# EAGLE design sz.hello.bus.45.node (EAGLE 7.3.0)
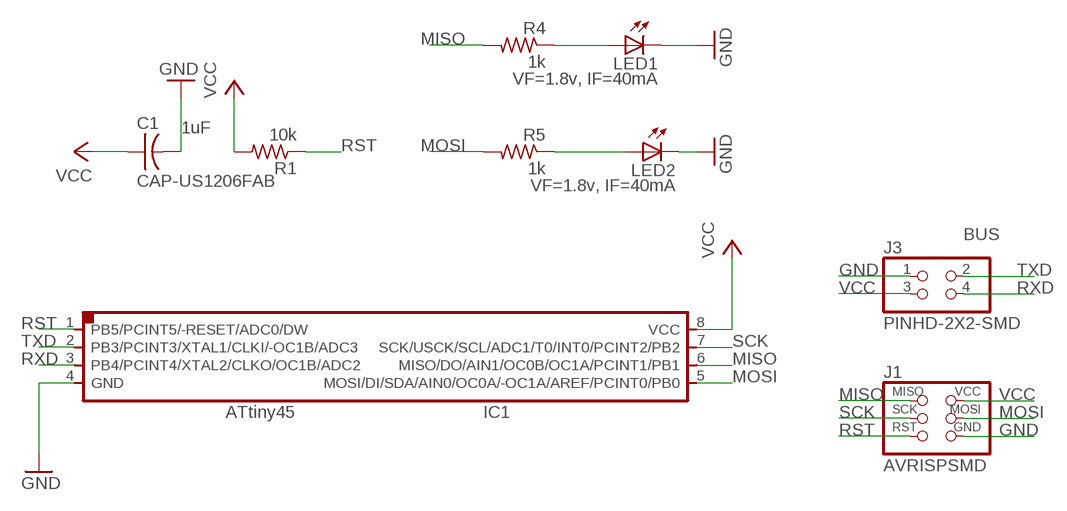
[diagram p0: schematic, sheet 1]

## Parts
C1  CAP-US1206FAB  [C1206FAB]
IC1  ATTINY45SI  [SOIC8]
J1  AVRISPSMD  [2X03SMD]
J3  PINHD-2X2-SMD  [2X02SMD]
LED1  VF=1.8v, IF=40mA  LEDSMT1206  [1206]
LED2  VF=1.8v, IF=40mA  LEDSMT1206  [1206]
R1  10k  RES-US1206FAB  [R1206FAB]
R4  1k  RES-US1206FAB  [R1206FAB]
R5  1k  RES-US1206FAB  [R1206FAB]

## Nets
GND: C1.2 IC1.4(GND) J1.6(GND) J3.1 LED1.C LED2.C
MISO: IC1.6(MISO/DO/AIN1/OC0B/OC1A/PCINT1/PB1) J1.1(MISO) R4.2
MOSI: IC1.5(MOSI/DI/SDA/AIN0/OC0A/-OC1A/AREF/PCINT0/PB0) J1.4(MOSI) R5.2
N$1: LED2.A R5.1
N$2: LED1.A R4.1
RST: IC1.1(PB5/PCINT5/-RESET/ADC0/DW) J1.5(RST) R1.1
RXD: IC1.3(PB4/PCINT4/XTAL2/CLKO/OC1B/ADC2) J3.4
SCK: IC1.7(SCK/USCK/SCL/ADC1/T0/INT0/PCINT2/PB2) J1.3(SCK)
TXD: IC1.2(PB3/PCINT3/XTAL1/CLKI/-OC1B/ADC3) J3.2
VCC: C1.1 IC1.8(VCC) J1.2(VCC) J3.3 R1.2

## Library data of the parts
C1 = fab:CAP-US; CAP: 1uF
IC1 = fab:ATTINY45
J1 = fab:AVRISP
J3 = fab:PINHD-2X2-SMD
LED1 LED2 = led:LED: LED
R1 R4 R5 = fab:RES-US: Resistor (US Symbol)

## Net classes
0 default: width 0.406 mm, drill 0.406 mm, clearance 0.457 mm

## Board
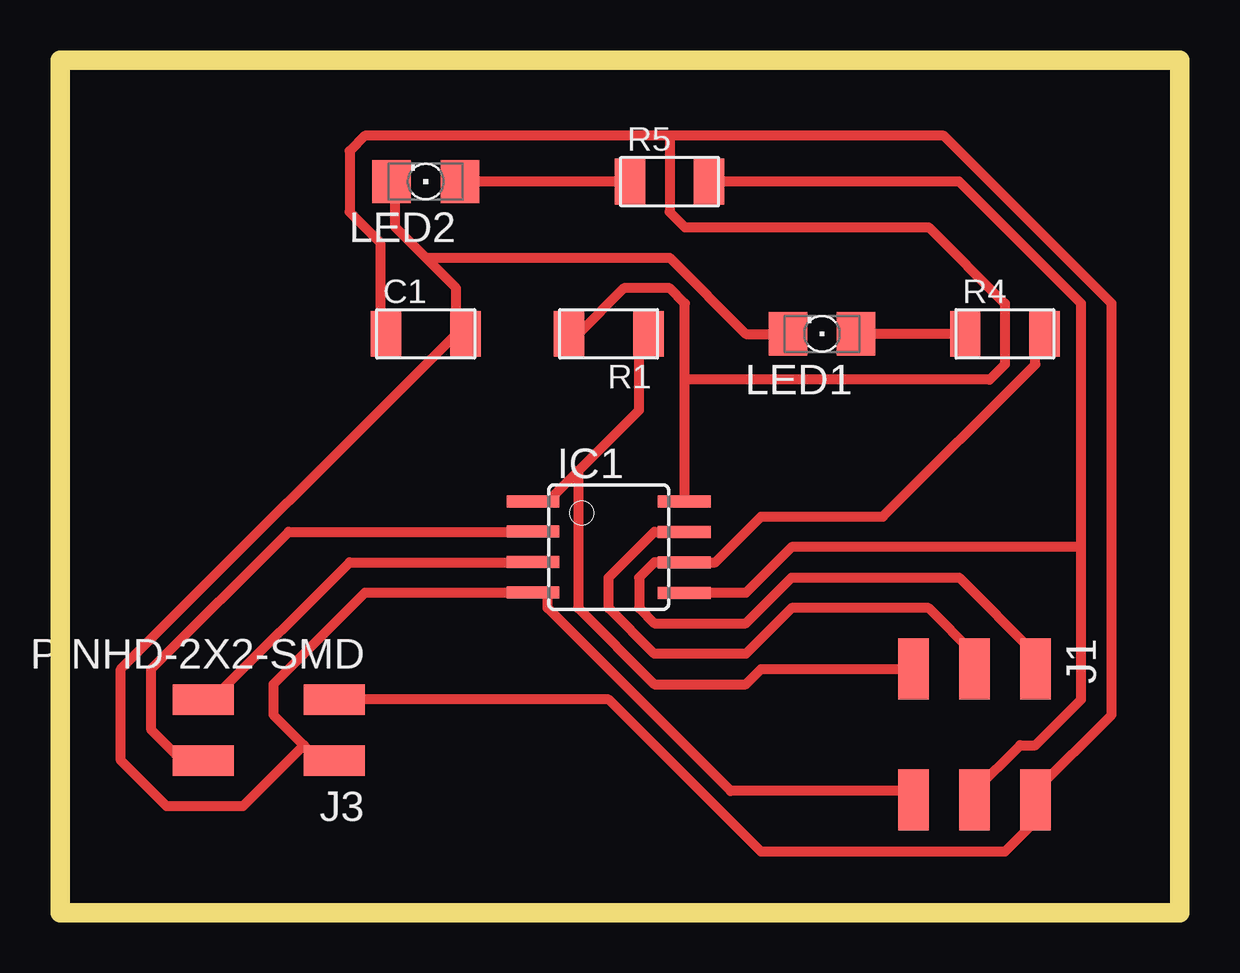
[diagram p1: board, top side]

Size 46.66 x 35.55 mm. Coordinates in mm from the lower left corner, seen from the top.
Outline: 0,0 46.66,0 46.66,35.55 0,35.55 0,0
Copper layers (1*16): Top 0.035mm / dielectric 1.5mm / Bottom 0.035mm
Design rules "default *": minimum track width 16mil, minimum drill 24mil, track to track 18mil, track to pad 18mil, pad to pad 8mil, via to via 8mil, smd to smd 8mil, copper to edge 40mil, drill to drill 8mil, minimum pad ring 10mil, minimum via ring 8mil, stop-mask expansion 4mil, vias tented up to drill 0mil, thermal gap 10mil

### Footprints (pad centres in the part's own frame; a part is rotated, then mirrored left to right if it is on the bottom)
C1206FAB = smd 1.27 x 1.905: 1 -1.651,0; 2 1.651,0
SOIC8 = smd 0.5 x 2.2: 1 -1.905,-3.154; 2 -0.645,-3.154; 3 0.625,-3.154; 4 1.895,-3.154; 5 1.905,3.154; 6 0.635,3.154; 7 -0.635,3.154; 8 -1.905,3.154
2X03SMD = smd 2.54 x 1.27: 1 -2.54,2.54; 2 2.92,2.54; 3 -2.54,0; 4 2.92,0; 5 -2.54,-2.54; 6 2.92,-2.54
2X02SMD = smd 2.54 x 1.27: 1 -2.54,1.27; 2 2.92,1.27; 3 -2.54,-1.27; 4 2.92,-1.27
1206 = smd 1.6 x 1.803: A -1.422,0; C 1.422,0
R1206FAB = smd 1.27 x 1.905: 1 -1.651,0; 2 1.651,0

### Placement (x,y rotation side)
C1  15.24,24.13 0 top
IC1  22.86,15.24 270 top
J1  38.1,7.62 270 top
J3  8.89,7.62 180 top
LED1  31.75,24.13 180 top
LED2  15.24,30.48 180 top
R1  22.86,24.13 180 top
R4  39.37,24.13 0 top
R5  25.4,30.48 0 top

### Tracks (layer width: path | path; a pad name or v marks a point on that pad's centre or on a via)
GND
  Top 0.406: 15.24,27.3 16.51,26.04 16.51,24.13 | 15.24,27.3 13.97,28.57 13.97,30.48 LED2.C | LED1.C 28.57,24.13 25.4,27.3 15.24,27.3 | J1.6 35.56,5.08 27.94,5.08 20.32,12.7 20.32,13.34 IC1.4 19.68,13.34 12.7,13.34 8.89,9.53 8.89,8.26 10.16,6.99 | J3.1 10.79,6.35 10.16,6.99 | 16.51,24.13 2.54,10.16 2.54,6.35 4.45,4.45 7.62,4.45 10.16,6.99 | 16.51,24.13 C1.2
MISO
  Top 0.406: R4.2 40.64,24.13 40.64,22.86 34.29,16.51 29.21,16.51 27.3,14.61 IC1.6 24.77,14.61 24.13,13.97 24.13,12.7 24.77,12.06 28.57,12.06 30.48,13.97 37.47,13.97 40.64,10.79 J1.1
MOSI
  Top 0.406: R5.2 37.47,30.48 42.55,25.4 42.55,15.24 | 42.55,15.24 42.55,8.89 40.64,6.99 40.01,6.99 38.1,5.08 J1.4 | IC1.5 28.57,13.34 30.48,15.24 42.55,15.24
N$1
  Top 0.406: R5.1 LED2.A
N$2
  Top 0.406: R4.1 LED1.A
RST
  Top 0.406: 21.59,18.41 20.32,17.14 IC1.1 | 21.59,18.41 24.13,20.95 24.13,24.13 R1.1 | J1.5 29.21,10.16 28.57,9.53 24.77,9.53 21.59,12.7 21.59,18.41
RXD
  Top 0.406: IC1.3 19.68,14.61 12.06,14.61 6.35,8.89 J3.4
SCK
  Top 0.406: IC1.7 24.77,15.88 22.86,13.97 22.86,12.7 24.77,10.79 28.57,10.79 30.48,12.7 36.2,12.7 38.1,10.79 J1.3
TXD
  Top 0.406: J3.2 5.08,6.35 3.81,7.62 3.81,10.16 9.53,15.88 19.68,15.88 IC1.2
VCC
  Top 0.406: 26.04,22.23 26.04,17.14 IC1.8 | 26.04,22.23 26.04,25.4 25.4,26.04 23.5,26.04 21.59,24.13 R1.2 | 25.4,32.38 36.83,32.38 43.82,25.4 43.82,8.26 40.64,5.08 J1.2 40.64,3.81 39.37,2.54 29.21,2.54 22.86,8.89 J3.3 | 25.4,32.38 12.7,32.38 12.06,31.75 12.06,29.21 13.33,27.94 13.33,24.13 C1.1 | 26.04,22.23 38.74,22.23 39.37,22.86 39.37,25.4 36.2,28.57 26.04,28.57 25.4,29.21 25.4,32.38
